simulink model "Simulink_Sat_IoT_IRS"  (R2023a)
settings: Solver=VariableStepAuto  StartTime=0.0  StopTime=10.0  RelTol=1e-3
model workspace (MAT data in the model file):
  Param : Simulink.Parameter (value not decoded)
  theta = [1 0.1 2 0.2 3 0.3 4 0.4]
libraries: commchan3 x2

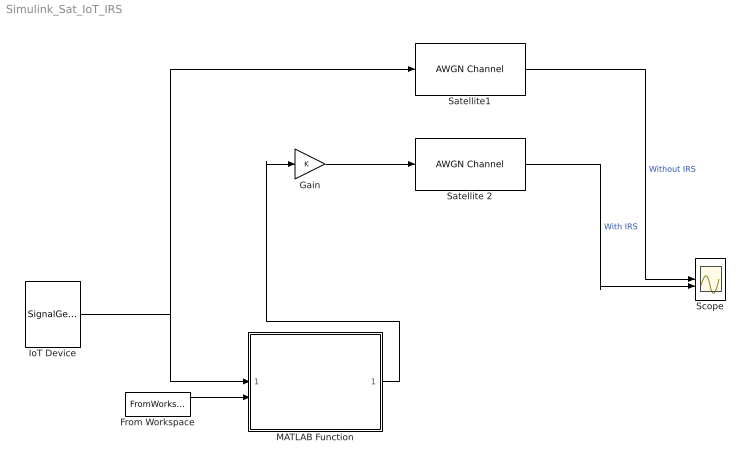
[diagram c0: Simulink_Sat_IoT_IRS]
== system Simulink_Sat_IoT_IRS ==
  From Workspace : FromWorkspace  VariableName=theta  OutDataTypeStr=double
  Gain : Gain
  IoT Device : SignalGenerator  Frequency=0.3  VectorParams1D=off
  MATLAB Function : MATLAB Function  TreatAsAtomicUnit=on
  Satellite 2 : commchan3/AWGN Channel  LegacyMode=off  NoiseMethod="Signal to noise ratio  (SNR)"  noiseMode="Signal to noise ratio  (SNR)"  EbNo=10  EsNo=10  SNR=20  BitsPerSymbol=1  SignalPower=10  SamplesPerSymbol=1  SymbolPeriod=1  VarianceSource=Parameter  Variance=1  RandomStream=Global stream  Seed=67  SimulateUsing=Interpreted execution
  Satellite1 : commchan3/AWGN Channel  LegacyMode=off  NoiseMethod="Signal to noise ratio  (SNR)"  noiseMode="Signal to noise ratio  (SNR)"  EbNo=10  EsNo=10  SNR=20  BitsPerSymbol=1  SignalPower=10  SamplesPerSymbol=1  SymbolPeriod=1  VarianceSource=Parameter  Variance=1  RandomStream=Global stream  Seed=67  SimulateUsing=Interpreted execution
  Scope : Scope  NumInputPorts=2
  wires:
  IoT Device/1 -> MATLAB Function/1(x), Satellite1/1
  Gain/1 -> Satellite 2/1
  MATLAB Function/1(y) -> Gain/1
  Satellite 2/1 -> Scope/2  "With IRS"
  From Workspace/1 -> MATLAB Function/2(theta)
  Satellite1/1 -> Scope/1  "Without IRS"

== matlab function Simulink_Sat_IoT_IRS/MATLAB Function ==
function y = irs_function(x, theta)
    % theta: Phase shifts for IRS elements
    % Define the theta vector 
    %theta = [0.1; 0.2; 0.3];
    % Inputs:
    % x: Incident signal
    % Outputs:
    % y: Reflected signal

    N = numel(theta); % Number of IRS elements

    y = zeros(size(x));
    for n = 1:N
        phase_shift = exp(1i * theta(n)); % Phase shift
        y = y + real(phase_shift * x);
    end
end
